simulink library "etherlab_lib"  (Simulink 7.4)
settings: Solver=ode45  SolverMode=SingleTasking  StartTime=0.0  StopTime=10.0  RelTol=1e-3
undefined symbols (not defined in the file or in its folder): ATD4, baumer_ecatencoder, bits, Boolean, BT, CoE, CW, DC, DI8DO8, Disabled, EK1100, EK1914, ekxxxx, EL1004, EL1262, EL1904, el1xxx, EL2004, EL2262, EL2535, el2535, EL2904, el2xxx, EL3002, EL3102, EL3201, EL3204, el320x_1, EL3255, EL3314, el331x, EL3356, el3356, EL3403, el3403, EL3602, el36x2, EL3702, el37x2, EL4002, el4xxx, EL5001, el500x, EL5021, el5021, EL5101, EL5152, El5152, EL51x1, el51xx, EL6001, el60xx, EL9110, el9xxx, EP1008, ep1xxx, EP2001, ep2xxx, EP3174, EP3182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
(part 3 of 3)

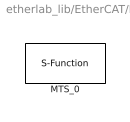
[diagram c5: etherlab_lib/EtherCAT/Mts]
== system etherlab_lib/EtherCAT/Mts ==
  MTS_0 : S-Function  FunctionName=ec_slave3  Parameters=Address, rv.SlaveConfig, rv.PortConfig, debug, tsample  SFunctionModules='ecrt_support'  EnableBusSupport=off  mask(MTS R-Series){master=0, index=1, model=1 Magnet, offset=[], invert=off, velocity_output=off, status_output=off, filter=off, tau=[], tsample=0, debug=0}
      mask prompts: index "Slave Index"; model "Device Model"; offset "Output Offset"; invert "Invert Position / Velocity"; velocity_output "Velocity Output"; status_output "Status Output"; filter "Output Filter"; tau "LPF Time Constant [s]"; tsample "Sample Time"
      mask help: MTS R-Series Position Senor Output 1: position vector (magnets 1-5) in meter Optional output 2: speed vector (magnets 1-5) in m/s Optional output 3: status vector (magnets 1-5)
      mask init:
      | Address = EtherCATSlave.formatAddress(master,index,tsample);
      | 
      | rv = mts_temposonics(model, offset, filter, tau, ...
      |                      invert, velocity_output, status_output);
      | 
      | rv.PortConfig.swap_io = EtherCATSlave.shouldSwapIoPorts();

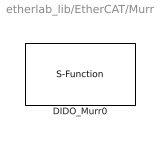
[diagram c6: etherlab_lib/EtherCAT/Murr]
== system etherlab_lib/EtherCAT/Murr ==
  DIDO_Murr0 : S-Function  LoadFcn=murr_dio().checkModelName()  FunctionName=ec_slave3  Parameters=Address,rv.SlaveConfig,rv.PortConfig,debug,tsample  SFunctionModules='ecrt_support'  EnableBusSupport=off  mask(Murr Impact67 EC){master=0, index=1, model=DI8DO8, revision=, vector=on, tsample=0, debug=0}
      mask prompts: index "Slave Index"; model "Device Model"; vector "Vector IO"; tsample "Sample Time (-1 for inherited)"
      mask help: Murr Impact67 EC Digital IO-Terminal
      mask init:
      | Address = EtherCATSlave.formatAddress(master,index,tsample);
      | 
      | rv = murr_dio(model).configure(vector);
      | 
      | if isfield(rv.PortConfig,'input')
      |     inputNames = {rv.PortConfig.input.portname};
      | else
      |     inputNames = {};
      | end
      | 
      | rv.PortConfig.swap_io = EtherCATSlave.shouldSwapIoPorts();
      | 
      | EtherCATSlave.setPortNames(...
      |     inputNames,...
      |     {rv.PortConfig.output.portname});
      | 
      | set_param(gcb,'AttributesFormatString',...
      |     sprintf('%s\nM:%i Idx:%s',model,master,mat2str(index)))

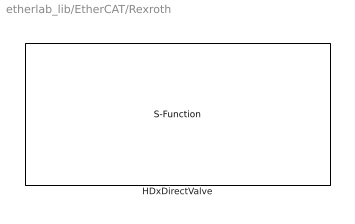
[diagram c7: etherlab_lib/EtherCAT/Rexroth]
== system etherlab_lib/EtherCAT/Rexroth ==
  HDxDirectValve : S-Function  LoadFcn=HDxDirectValve().checkModelName  FunctionName=ec_slave3  Parameters=Address,rv.SlaveConfig,rv.PortConfig,debug,tsample  SFunctionModules='ecrt_support'  EnableBusSupport=off  mask(HDxDirectValve){master=0, index=1, model=HDx20V12+ CoE, revision=, vector=on, tsample=0, debug=0, firmware_flavour=HDB (IAC), analogInRange1=Disabled, analogInRange2=Disabled, analogInRange3=Disabled, analogInRange4=Disabled}
      mask prompts: index "Slave Index"; model "Device Model"; vector "Vector Outputs"; tsample "Sample Time"; debug "Debug Level"; firmware_flavour "Firmware Flavour"; analogInRange1 "Analog Input 1"; analogInRange2 "Analog Input 2"; analogInRange3 "Analog Input 3"; analogInRange4 "Analog Input 4"
      mask help: Rexroth HDB or HDE EtherCAT Valve running CiA408 Fluid Power Profile
      mask init:
      | Address = EtherCATSlave.formatAddress(master,index,tsample);
      | 
      | analogInputs = [
      |     analogInRange1;
      |     analogInRange2;
      |     analogInRange3;
      |     analogInRange4;
      | ];
      | 
      | rv = HDxDirectValve(model).configure(firmware_flavour, analogInputs);
      | rv.PortConfig.swap_io = EtherCATSlave.shouldSwapIoPorts();
      | 
      | inp = arrayfun(@(x) x.portname, rv.PortConfig.input, 'UniformOutput', false);
      | outp = arrayfun(@(x) x.portname, rv.PortConfig.output, 'UniformOutput', false);
      | 
      | EtherCATSlave.setPortNames(inp, outp);
      | 
      | set_param(gcb,'AttributesFormatString',...
      |     sprintf('%s\nM:%i Idx:%s',...
      |             model,master,mat2str(index)))

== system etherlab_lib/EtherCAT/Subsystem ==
